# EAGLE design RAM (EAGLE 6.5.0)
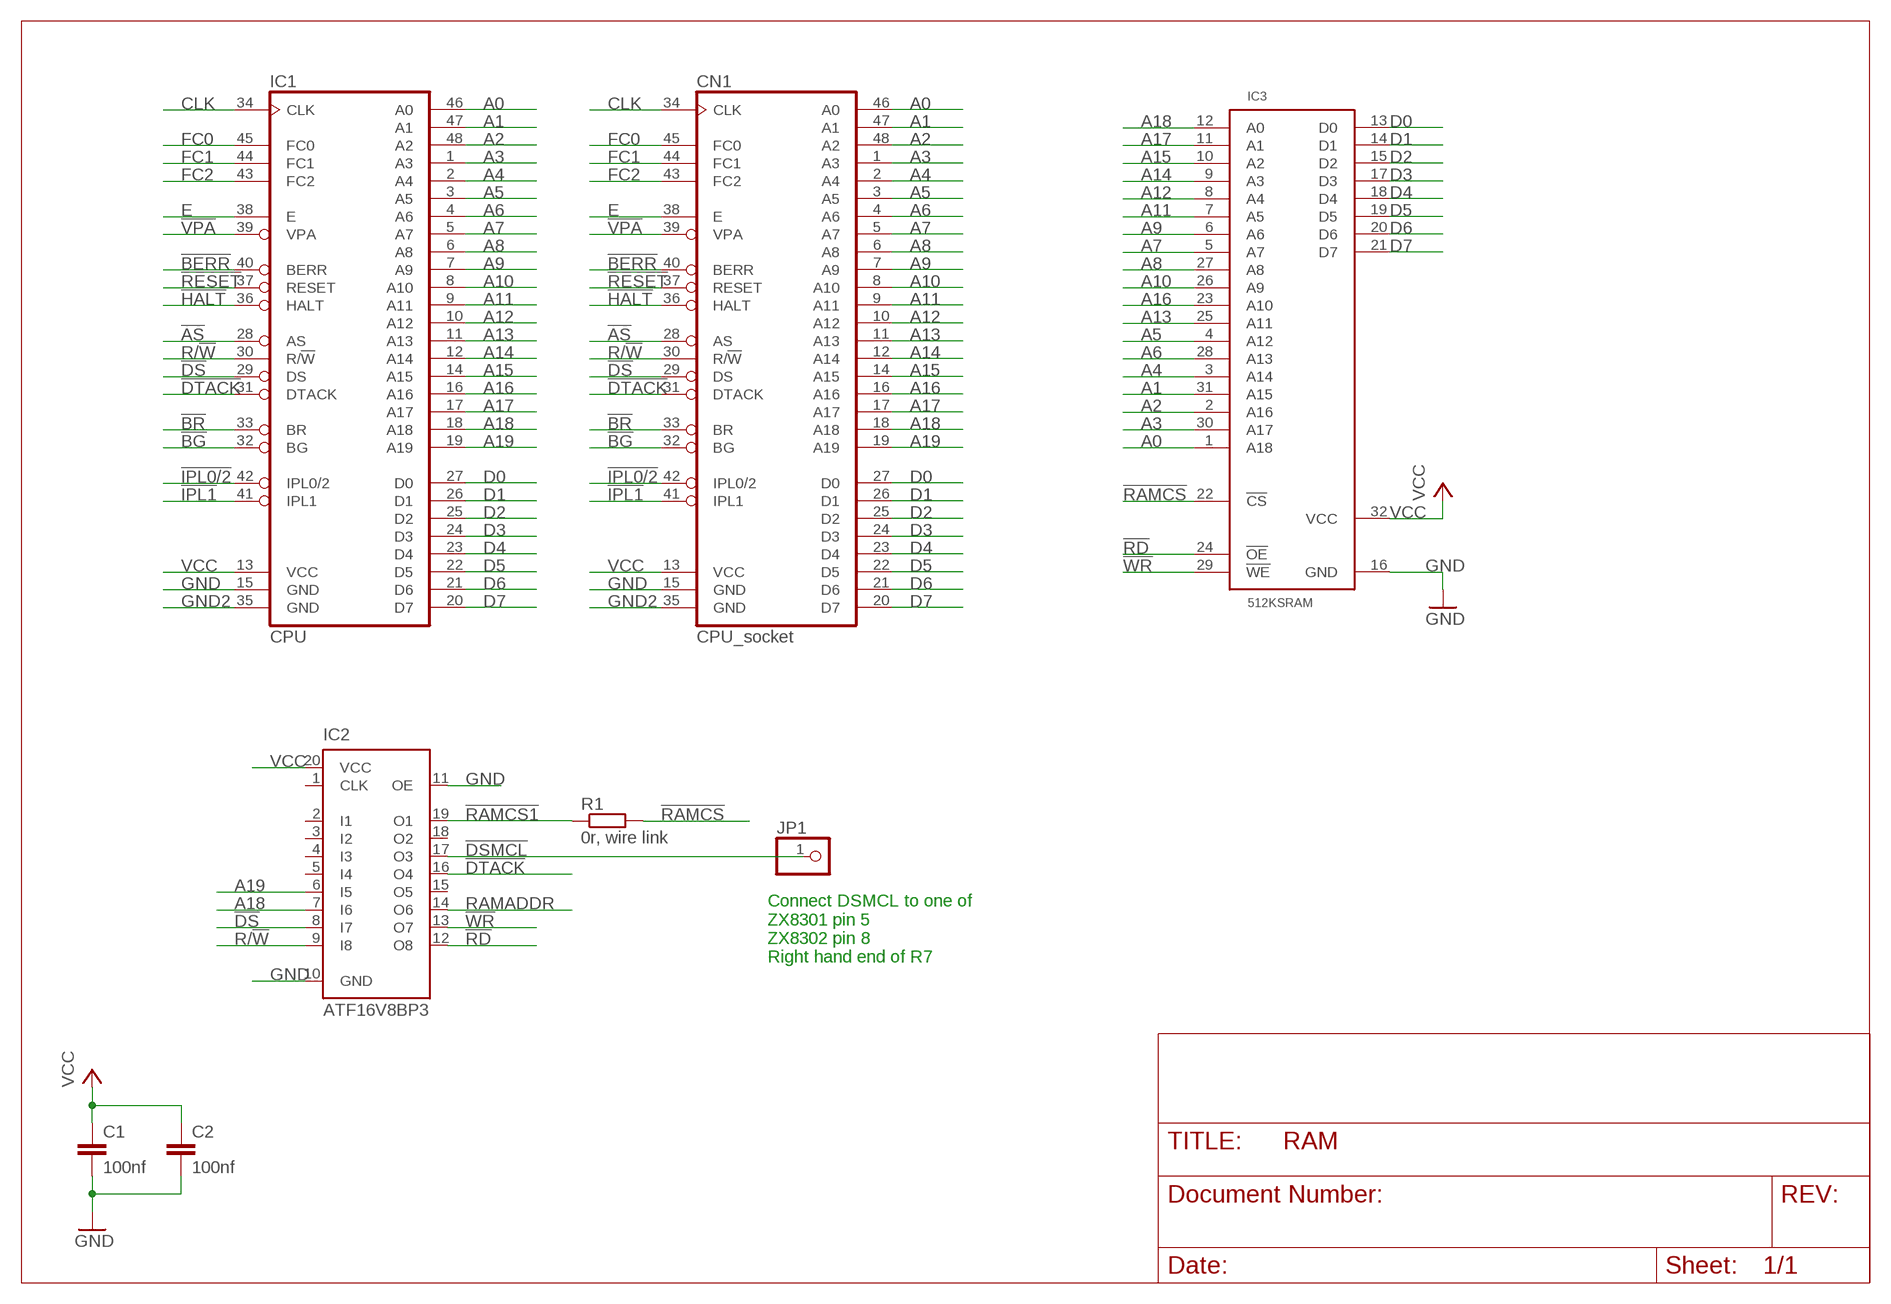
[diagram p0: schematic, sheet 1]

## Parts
C1  100nf  C-EU050-024X044  [C050-024X044]
C2  100nf  C-EU050-024X044  [C050-024X044]
CN1  CPU_socket  MC68008P  [DIL48]
IC1  CPU  MC68008P-1MM-HOLES  [DIL48-1MM]
IC2  ATF16V8BP3  [DIL20]
IC3  512KSRAM  [DIL32]
JP1  PINHD-1X1  [1X01]
R1  0r, wire link  R-EU_0207/10  [0207/10]

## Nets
!AS: CN1.28(AS) IC1.28(AS)
!BERR: CN1.40(BERR) IC1.40(BERR)
!BG: CN1.32(BG) IC1.32(BG)
!BR: CN1.33(BR) IC1.33(BR)
!DS: CN1.29(DS) IC1.29(DS) IC2.8(I7)
!DSMCL: IC2.17(O3) JP1.1
!DTACK: CN1.31(DTACK) IC1.31(DTACK) IC2.16(O4)
!HALT: CN1.36(HALT) IC1.36(HALT)
!IPL0/2: CN1.42(IPL0/2) IC1.42(IPL0/2)
!IPL1: CN1.41(IPL1) IC1.41(IPL1)
!RAMCS: IC3.22(!CS) R1.2
!RAMCS1: IC2.19(O1) R1.1
!RD: IC2.12(O8) IC3.24(!OE)
!RESET: CN1.37(RESET) IC1.37(RESET)
!VPA: CN1.39(VPA) IC1.39(VPA)
!WR: IC2.13(O7) IC3.29(!WE)
A0: CN1.46(A0) IC1.46(A0) IC3.1(A18)
A1: CN1.47(A1) IC1.47(A1) IC3.31(A15)
A2: CN1.48(A2) IC1.48(A2) IC3.2(A16)
A3: CN1.1(A3) IC1.1(A3) IC3.30(A17)
A4: CN1.2(A4) IC1.2(A4) IC3.3(A14)
A5: CN1.3(A5) IC1.3(A5) IC3.4(A12)
A6: CN1.4(A6) IC1.4(A6) IC3.28(A13)
A7: CN1.5(A7) IC1.5(A7) IC3.5(A7)
A8: CN1.6(A8) IC1.6(A8) IC3.27(A8)
A9: CN1.7(A9) IC1.7(A9) IC3.6(A6)
A10: CN1.8(A10) IC1.8(A10) IC3.26(A9)
A11: CN1.9(A11) IC1.9(A11) IC3.7(A5)
A12: CN1.10(A12) IC1.10(A12) IC3.8(A4)
A13: CN1.11(A13) IC1.11(A13) IC3.25(A11)
A14: CN1.12(A14) IC1.12(A14) IC3.9(A3)
A15: CN1.14(A15) IC1.14(A15) IC3.10(A2)
A16: CN1.16(A16) IC1.16(A16) IC3.23(A10)
A17: CN1.17(A17) IC1.17(A17) IC3.11(A1)
A18: CN1.18(A18) IC1.18(A18) IC2.7(I6) IC3.12(A0)
A19: CN1.19(A19) IC1.19(A19) IC2.6(I5)
CLK: CN1.34(CLK) IC1.34(CLK)
D0: CN1.27(D0) IC1.27(D0) IC3.13(D0)
D1: CN1.26(D1) IC1.26(D1) IC3.14(D1)
D2: CN1.25(D2) IC1.25(D2) IC3.15(D2)
D3: CN1.24(D3) IC1.24(D3) IC3.17(D3)
D4: CN1.23(D4) IC1.23(D4) IC3.18(D4)
D5: CN1.22(D5) IC1.22(D5) IC3.19(D5)
D6: CN1.21(D6) IC1.21(D6) IC3.20(D6)
D7: CN1.20(D7) IC1.20(D7) IC3.21(D7)
E: CN1.38(E) IC1.38(E)
FC0: CN1.45(FC0) IC1.45(FC0)
FC1: CN1.44(FC1) IC1.44(FC1)
FC2: CN1.43(FC2) IC1.43(FC2)
GND: C1.2 C2.2 CN1.15(GND) IC1.15(GND) IC2.10(GND) IC2.11(OE) IC3.16(GND)
GND2: CN1.35(GND) IC1.35(GND)
R/!W!: CN1.30(R/!W) IC1.30(R/!W) IC2.9(I8)
RAMADDR: IC2.14(O6)
VCC: C1.1 C2.1 CN1.13(VCC) IC1.13(VCC) IC2.20(VCC) IC3.32(VCC)
Unconnected: IC2.1(CLK) IC2.2(I1) IC2.3(I2) IC2.4(I3) IC2.5(I4) IC2.15(O5) IC2.18(O2)

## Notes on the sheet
- Connect DSMCL to one of 
  ZX8301 pin 5
  ZX8302 pin 8
  Right hand end of R7

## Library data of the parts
C1 C2 = rcl:C-EU: CAPACITOR, European symbol
CN1 = Con-Sinclair:MC68008P: 68xxx PROCESSOR; OC_FARNELL: unknown; OC_NEWARK: unknown
IC1 = Con-Sinclair:MC68008P: 68xxx PROCESSOR
IC2 = atmel:ATF16V8B: High perfomance CMOS (electrically erasable) programmable logic device (PLD) ABLE-Atmel-ABEL - P18V8R, P16V8C, P16V8AS, P17V8 COPL Atmel-WinCUPL - G16V8MS, G16V8MA, G16V8AS, G16V8 LOG/IC - GAL16V8_R, GAL16V8_G7, GAL16V8_C), GAL16V8 Tango-PLD - G16V8R, G16V8C, G16V8AS, G16V8 Source: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; MPN: ATF16V8CZ-15PU; OC_FARNELL: 1551768; OC_NEWARK: 94M6254
IC3 = Rom-Ram:512KSRAM: 512K x 8 SRAM
JP1 = pinhead-round:PINHD-1X1: PIN HEADER
R1 = rcl:R-EU_: RESISTOR, European symbol

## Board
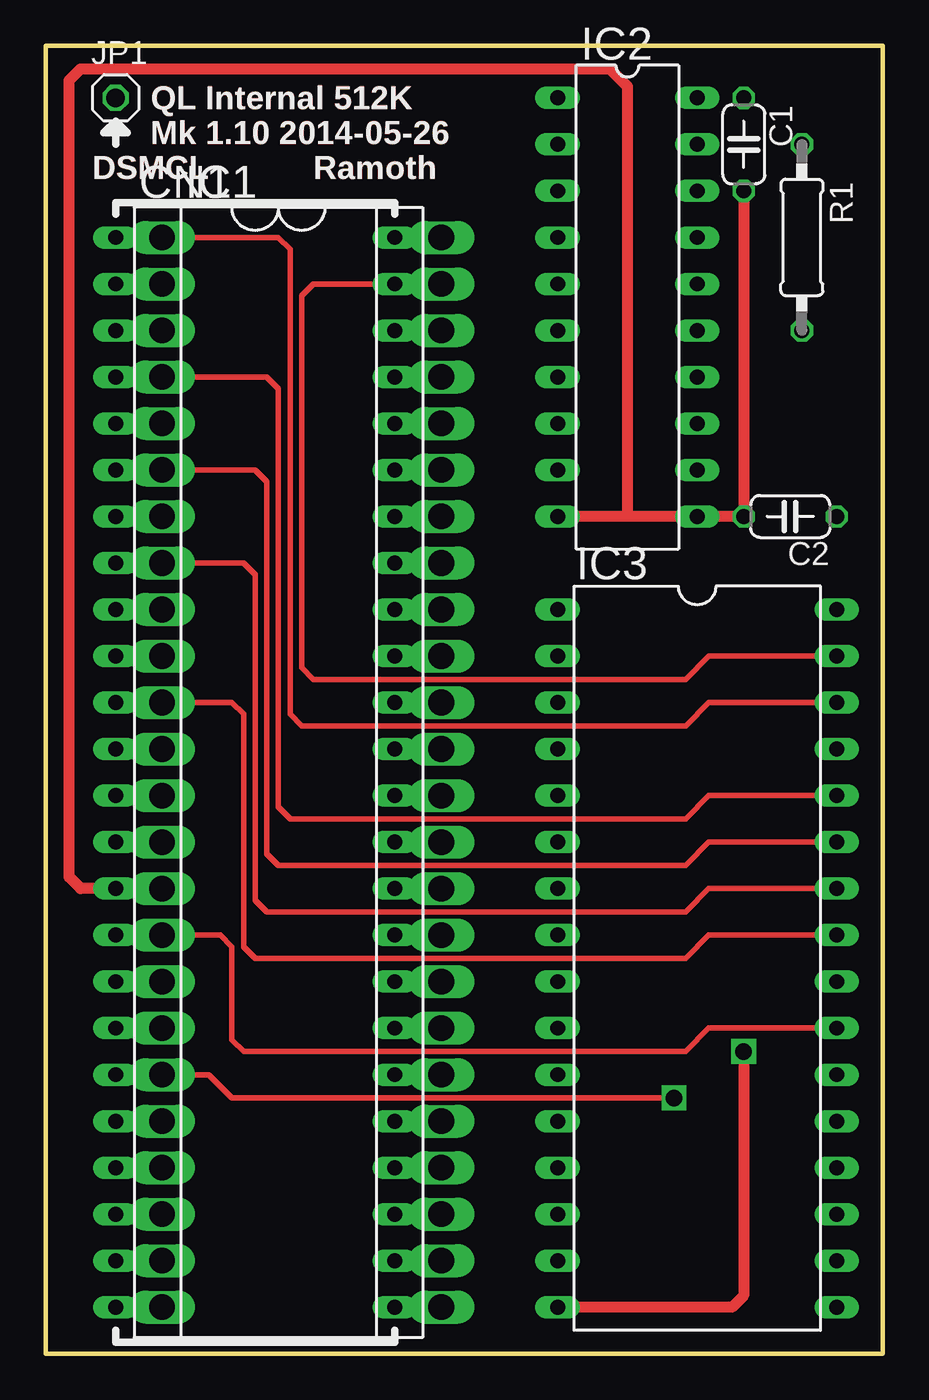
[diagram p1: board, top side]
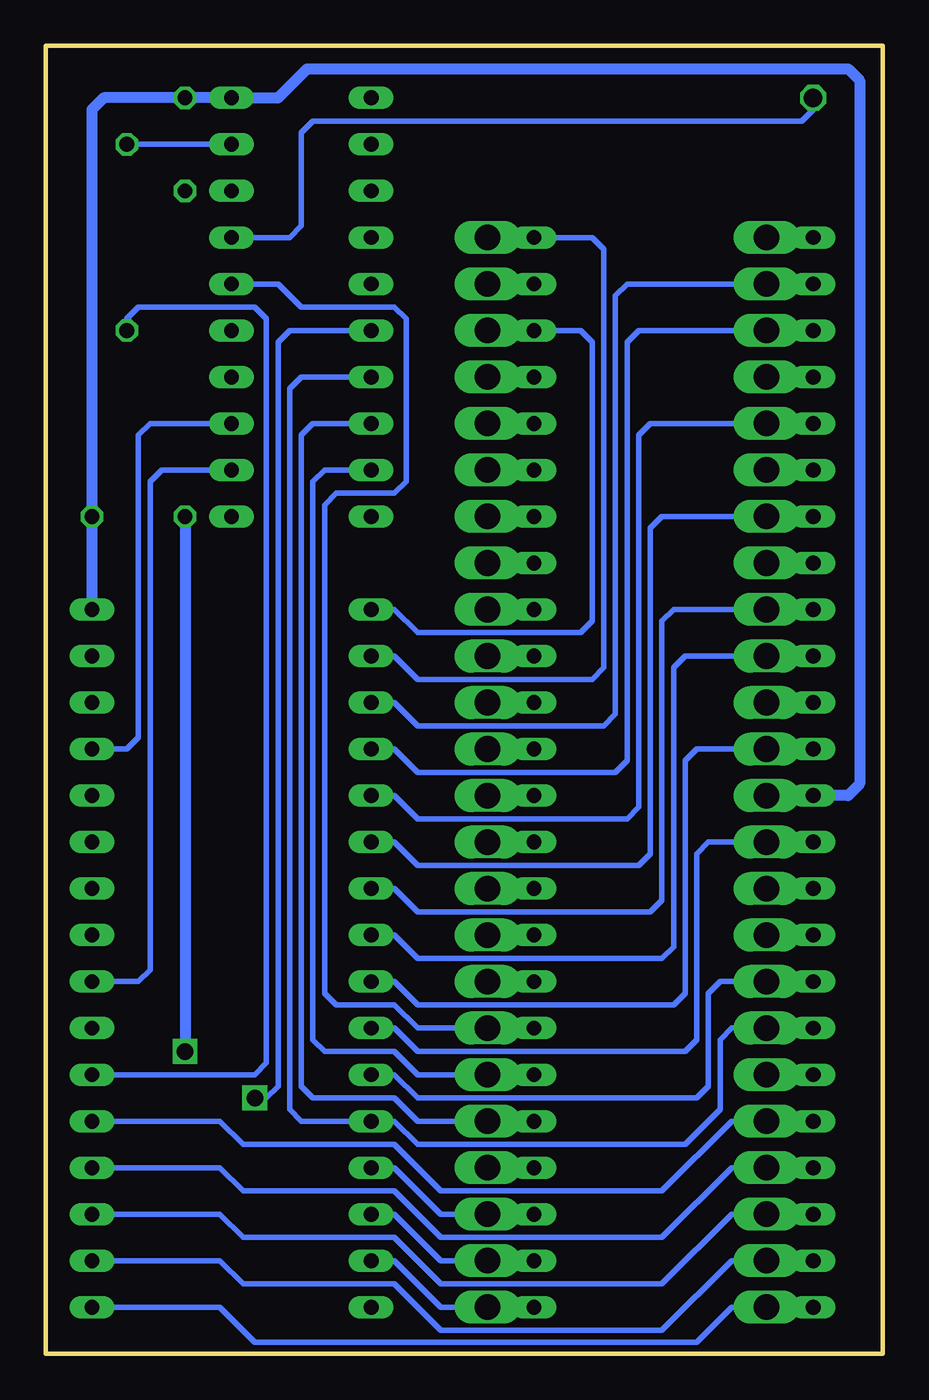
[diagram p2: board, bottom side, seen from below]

Size 45.7 x 71.42 mm. Coordinates in mm from the lower left corner, seen from the top.
Outline: 0,0 45.7,0 45.7,71.42 0,71.42 0,0
Copper layers (1*16): Top 0.035mm / dielectric 1.5mm / Bottom 0.035mm
Design rules "qimi *": minimum track width 10mil, minimum drill 24mil, track to track 8mil, track to pad 8mil, pad to pad 8mil, via to via 8mil, smd to smd 8mil, copper to edge 40mil, drill to drill 8mil, minimum pad ring 8mil, minimum via ring 8mil, stop-mask expansion 4mil, vias tented up to drill 0mil, thermal gap 10mil

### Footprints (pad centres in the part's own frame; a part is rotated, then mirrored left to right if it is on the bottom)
C050-024X044 = drill 0.813 octagon: 1 -2.54,0; 2 2.54,0
DIL48 = drill 0.813 long: 1 -29.21,-7.62; 2 -26.67,-7.62; 3 -24.13,-7.62; 4 -21.59,-7.62; 5 -19.05,-7.62; 6 -16.51,-7.62; 7 -13.97,-7.62; 8 -11.43,-7.62; 9 -8.89,-7.62; 10 -6.35,-7.62; 11 -3.81,-7.62; 12 -1.27,-7.62; 13 1.27,-7.62; 14 3.81,-7.62; 15 6.35,-7.62; 16 8.89,-7.62; 17 11.43,-7.62; 18 13.97,-7.62; 19 16.51,-7.62; 20 19.05,-7.62; 21 21.59,-7.62; 22 24.13,-7.62; 23 26.67,-7.62; 24 29.21,-7.62; 25 29.21,7.62; 26 26.67,7.62; 27 24.13,7.62; 28 21.59,7.62; 29 19.05,7.62; 30 16.51,7.62; 31 13.97,7.62; 32 11.43,7.62; 33 8.89,7.62; 34 6.35,7.62; 35 3.81,7.62; 36 1.27,7.62; 37 -1.27,7.62; 38 -3.81,7.62; 39 -6.35,7.62; 40 -8.89,7.62; 41 -11.43,7.62; 42 -13.97,7.62; 43 -16.51,7.62; 44 -19.05,7.62; 45 -21.59,7.62; 46 -24.13,7.62; 47 -26.67,7.62; 48 -29.21,7.62
DIL48-1MM = drill 1.4 pad 1.676 long: 1 -29.21,-7.62; 2 -26.67,-7.62; 3 -24.13,-7.62; 4 -21.59,-7.62; 5 -19.05,-7.62; 6 -16.51,-7.62; 7 -13.97,-7.62; 8 -11.43,-7.62; 9 -8.89,-7.62; 10 -6.35,-7.62; 11 -3.81,-7.62; 12 -1.27,-7.62; 13 1.27,-7.62; 14 3.81,-7.62; 15 6.35,-7.62; 16 8.89,-7.62; 17 11.43,-7.62; 18 13.97,-7.62; 19 16.51,-7.62; 20 19.05,-7.62; 21 21.59,-7.62; 22 24.13,-7.62; 23 26.67,-7.62; 24 29.21,-7.62; 25 29.21,7.62; 26 26.67,7.62; 27 24.13,7.62; 28 21.59,7.62; 29 19.05,7.62; 30 16.51,7.62; 31 13.97,7.62; 32 11.43,7.62; 33 8.89,7.62; 34 6.35,7.62; 35 3.81,7.62; 36 1.27,7.62; 37 -1.27,7.62; 38 -3.81,7.62; 39 -6.35,7.62; 40 -8.89,7.62; 41 -11.43,7.62; 42 -13.97,7.62; 43 -16.51,7.62; 44 -19.05,7.62; 45 -21.59,7.62; 46 -24.13,7.62; 47 -26.67,7.62; 48 -29.21,7.62
DIL20 = drill 0.813 long: 1 -11.43,-3.81; 2 -8.89,-3.81; 3 -6.35,-3.81; 4 -3.81,-3.81; 5 -1.27,-3.81; 6 1.27,-3.81; 7 3.81,-3.81; 8 6.35,-3.81; 9 8.89,-3.81; 10 11.43,-3.81; 11 11.43,3.81; 12 8.89,3.81; 13 6.35,3.81; 14 3.81,3.81; 15 1.27,3.81; 16 -1.27,3.81; 17 -3.81,3.81; 18 -6.35,3.81; 19 -8.89,3.81; 20 -11.43,3.81
DIL32 = drill 0.813 long: 1 -19.05,-7.62; 2 -16.51,-7.62; 3 -13.97,-7.62; 4 -11.43,-7.62; 5 -8.89,-7.62; 6 -6.35,-7.62; 7 -3.81,-7.62; 8 -1.27,-7.62; 9 1.27,-7.62; 10 3.81,-7.62; 11 6.35,-7.62; 12 8.89,-7.62; 13 11.43,-7.62; 14 13.97,-7.62; 15 16.51,-7.62; 16 19.05,-7.62; 17 19.05,7.62; 18 16.51,7.62; 19 13.97,7.62; 20 11.43,7.62; 21 8.89,7.62; 22 6.35,7.62; 23 3.81,7.62; 24 1.27,7.62; 25 -1.27,7.62; 26 -3.81,7.62; 27 -6.35,7.62; 28 -8.89,7.62; 29 -11.43,7.62; 30 -13.97,7.62; 31 -16.51,7.62; 32 -19.05,7.62
1X01 = drill 1.016 octagon: 1 0,0
0207/10 = drill 0.813 octagon: 1 -5.08,0; 2 5.08,0

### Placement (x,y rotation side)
C1  38.1,66.04 270 top
C2  40.64,45.72 180 top
CN1  11.43,31.75 270 top
IC1  13.97,31.75 270 top
IC2  31.75,57.15 270 top
IC3  35.56,21.59 270 top
JP1  3.81,68.58 0 top
R1  41.27,60.96 270 top

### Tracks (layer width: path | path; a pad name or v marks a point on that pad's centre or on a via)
!AS
  Top 0.254: CN1.28 IC1.28
!BERR
  Top 0.254: CN1.40 IC1.40
!BG
  Top 0.254: CN1.32 IC1.32
!BR
  Top 0.254: CN1.33 IC1.33
!DS
  Top 0.254: CN1.29 IC1.29
  Bottom 0.305: IC1.29 25.4,12.7 26.67,13.97 31.11,13.97 31.75,14.61 31.75,50.16 31.11,50.8 IC2.8
!DSMCL
  Bottom 0.305: JP1.1 3.81,67.94 4.45,67.31 31.11,67.31 31.75,66.67 31.75,61.59 32.38,60.96 IC2.17
!DTACK
  Top 0.254: CN1.31 IC1.31
  Bottom 0.305: IC2.16 33.02,58.42 31.75,57.15 26.67,57.15 26.04,56.52 26.04,47.62 26.67,46.99 29.84,46.99 30.48,46.35 30.48,19.68 29.84,19.05 26.67,19.05 25.4,17.78 IC1.31
!HALT
  Top 0.254: CN1.36 IC1.36
!IPL0/2
  Top 0.254: CN1.42 IC1.42
!IPL1
  Top 0.254: CN1.41 IC1.41
!RAMCS
  Bottom 0.305: R1.2 41.27,56.52 40.64,57.15 34.29,57.15 33.66,56.52 33.66,15.88 34.29,15.24 IC3.22
!RAMCS1
  Bottom 0.305: IC2.19 R1.1
!RD
  Bottom 0.305: IC2.12 39.37,48.26 40.01,47.62 40.01,20.95 40.64,20.32 IC3.24
!RESET
  Top 0.254: CN1.37 IC1.37
!VPA
  Top 0.254: CN1.39 IC1.39
!WR
  Bottom 0.305: IC2.13 40.01,50.8 40.64,50.16 40.64,33.66 41.27,33.02 IC3.29
A0
  Top 0.254: CN1.46 IC1.46
  Bottom 0.305: IC3.1 26.67,40.64 25.4,39.37 16.51,39.37 15.88,40.01 15.88,55.24 16.51,55.88 IC1.46
A1
  Top 0.254: CN1.47 IC1.47
  Top 0.305: IC3.31 36.2,38.1 34.92,36.83 14.61,36.83 13.97,37.47 13.97,57.78 14.61,58.42 IC1.47
A2
  Top 0.254: CN1.48 IC1.48
  Bottom 0.305: IC3.2 26.67,38.1 25.4,36.83 15.88,36.83 15.24,37.47 15.24,60.33 15.88,60.96 IC1.48
A3
  Top 0.254: CN1.1 IC1.1
  Top 0.305: CN1.1 12.7,60.96 13.34,60.33 13.34,34.92 13.97,34.29 34.92,34.29 36.2,35.56 IC3.30
A4
  Top 0.254: CN1.2 IC1.2
  Bottom 0.305: CN1.2 13.97,58.42 14.61,57.78 14.61,34.92 15.24,34.29 25.4,34.29 26.67,35.56 IC3.3
A5
  Top 0.254: CN1.3 IC1.3
  Bottom 0.305: CN1.3 13.34,55.88 13.97,55.24 13.97,32.38 14.61,31.75 25.4,31.75 26.67,33.02 IC3.4
A6
  Top 0.254: CN1.4 IC1.4
  Top 0.305: CN1.4 12.06,53.34 12.7,52.7 12.7,29.84 13.34,29.21 34.92,29.21 36.2,30.48 IC3.28
A7
  Top 0.254: CN1.5 IC1.5
  Bottom 0.305: CN1.5 12.7,50.8 13.34,50.16 13.34,29.84 13.97,29.21 25.4,29.21 26.67,30.48 IC3.5
A8
  Top 0.254: CN1.6 IC1.6
  Top 0.305: CN1.6 11.43,48.26 12.06,47.62 12.06,27.3 12.7,26.67 34.92,26.67 36.2,27.94 IC3.27
A9
  Top 0.254: CN1.7 IC1.7
  Bottom 0.305: CN1.7 12.06,45.72 12.7,45.09 12.7,27.3 13.34,26.67 25.4,26.67 26.67,27.94 IC3.6
A10
  Top 0.254: CN1.8 IC1.8
  Top 0.305: CN1.8 10.79,43.18 11.43,42.55 11.43,24.77 12.06,24.13 34.92,24.13 36.2,25.4 IC3.26
A11
  Top 0.254: CN1.9 IC1.9
  Bottom 0.305: CN1.9 11.43,40.64 12.06,40.01 12.06,24.77 12.7,24.13 25.4,24.13 26.67,25.4 IC3.7
A12
  Top 0.254: CN1.10 IC1.10
  Bottom 0.305: CN1.10 10.79,38.1 11.43,37.47 11.43,22.23 12.06,21.59 25.4,21.59 26.67,22.86 IC3.8
A13
  Top 0.254: CN1.11 IC1.11
  Top 0.305: CN1.11 10.16,35.56 10.79,34.92 10.79,22.23 11.43,21.59 34.92,21.59 36.2,22.86 IC3.25
A14
  Top 0.254: CN1.12 IC1.12
  Bottom 0.305: CN1.12 10.16,33.02 10.79,32.38 10.79,19.68 11.43,19.05 25.4,19.05 26.67,20.32 IC3.9
A15
  Top 0.254: CN1.14 IC1.14
  Bottom 0.305: CN1.14 9.53,27.94 10.16,27.3 10.16,17.14 10.79,16.51 25.4,16.51 26.67,17.78 IC3.10
A16
  Top 0.254: CN1.16 IC1.16
  Top 0.305: CN1.16 9.53,22.86 10.16,22.23 10.16,17.14 10.79,16.51 34.92,16.51 36.2,17.78 IC3.23
A17
  Top 0.254: CN1.17 IC1.17
  Bottom 0.305: CN1.17 8.89,20.32 9.53,19.68 9.53,14.61 10.16,13.97 25.4,13.97 26.67,15.24 IC3.11
A18
  Top 0.254: CN1.18 IC1.18
  Bottom 0.305: IC1.18 8.26,17.78 8.89,17.14 8.89,13.34 10.79,11.43 25.4,11.43 26.67,12.7 IC3.12 31.75,12.7 32.38,13.34 32.38,52.7 31.75,53.34 IC2.7
A19  (via drill 0.9)
  Top 0.254: CN1.19 IC1.19
  Top 0.305: IC1.19 8.89,15.24 10.16,13.97 v34.29,13.97
  Bottom 0.305: v34.29,13.97 33.66,13.97 33.02,14.61 33.02,55.24 32.38,55.88 IC2.6
CLK
  Top 0.254: CN1.34 IC1.34
D0
  Top 0.254: CN1.27 IC1.27
  Bottom 0.305: IC3.13 26.67,10.16 24.13,7.62 IC1.27
D1
  Top 0.254: CN1.26 IC1.26
  Bottom 0.305: IC3.14 26.67,7.62 24.13,5.08 IC1.26
D2
  Top 0.254: CN1.25 IC1.25
  Bottom 0.305: IC3.15 26.67,5.08 24.13,2.54 IC1.25
D3
  Top 0.254: CN1.24 IC1.24
  Bottom 0.305: CN1.24 8.26,2.54 10.16,0.64 34.29,0.64 36.2,2.54 IC3.17
D4
  Top 0.254: CN1.23 IC1.23
  Bottom 0.305: CN1.23 8.26,5.08 12.06,1.27 24.13,1.27 26.67,3.81 34.92,3.81 36.2,5.08 IC3.18
D5
  Top 0.254: CN1.22 IC1.22
  Bottom 0.305: CN1.22 8.26,7.62 12.06,3.81 24.13,3.81 26.67,6.35 34.92,6.35 36.2,7.62 IC3.19
D6
  Top 0.254: CN1.21 IC1.21
  Bottom 0.305: CN1.21 8.26,10.16 12.06,6.35 24.13,6.35 26.67,8.89 34.92,8.89 36.2,10.16 IC3.20
D7
  Top 0.254: CN1.20 IC1.20
  Bottom 0.305: CN1.20 8.26,12.7 12.06,8.89 24.13,8.89 26.67,11.43 34.92,11.43 36.2,12.7 IC3.21
E
  Top 0.254: CN1.38 IC1.38
FC0
  Top 0.254: CN1.45 IC1.45
FC1
  Top 0.254: CN1.44 IC1.44
FC2
  Top 0.254: CN1.43 IC1.43
GND  (via drill 0.9)
  Top 0.254: CN1.15 IC1.15
  Top 0.61: C1.2 C2.2 IC2.11 31.75,45.72 | 31.75,45.72 IC2.10 | v38.1,16.51 38.1,3.17 37.47,2.54 IC3.16 | IC1.15 1.91,25.4 1.27,26.04 1.27,69.53 1.91,70.17 30.8,70.17 31.75,69.22 31.75,45.72
  Bottom 0.61: C2.2 v38.1,16.51
GND2
  Top 0.254: CN1.35 IC1.35
N$1
  Top 0.406: 3.81,1.27 3.81,0.64 19.05,0.64 19.05,1.27
N$2
  Top 0.406: 3.81,62.23 3.81,62.87 19.05,62.87 19.05,62.23
N$3
  Top 0.406: 3.81,66.04 3.81,67.31 | 3.81,67.31 4.45,66.67 3.17,66.67 3.81,67.31
R/!W!
  Top 0.254: CN1.30 IC1.30
  Bottom 0.305: IC2.9 30.48,48.26 31.11,47.62 31.11,17.14 30.48,16.51 26.67,16.51 25.4,15.24 IC1.30
VCC
  Top 0.254: CN1.13 IC1.13
  Bottom 0.61: IC3.32 C2.1 43.18,67.94 42.55,68.58 C1.1 IC2.20 33.02,68.58 31.43,70.17 1.91,70.17 1.27,69.53 1.27,31.11 1.91,30.48 CN1.13

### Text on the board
Top: QL Internal 512K | Mk 1.10 2014-05-26 | DSMCL | Ramoth
tPlace: QL Internal 512K | Mk 1.10 2014-05-26 | DSMCL | Ramoth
